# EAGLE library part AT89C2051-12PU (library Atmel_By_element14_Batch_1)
Microcontroller
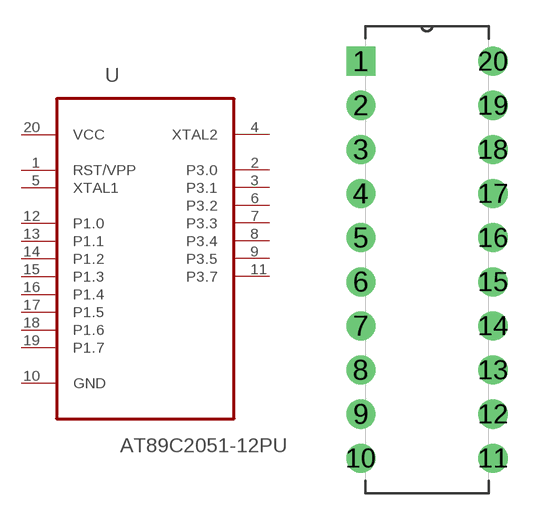
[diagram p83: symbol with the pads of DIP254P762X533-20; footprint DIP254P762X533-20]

Designator prefix U

## AT89C2051-12PU (MPN: AT89C2051-12PU; OC_FARNELL: 1699389; OC_NEWARK: 68T4860; PACKAGE: DIP-20; SUPPLIER: ATMEL)  [DIP254P762X533-20]
1  RST/VPP  in
2  P3.0
3  P3.1
4  XTAL2  out
5  XTAL1  in
6  P3.2
7  P3.3
8  P3.4
9  P3.5
10  GND  pas
11  P3.7
12  P1.0
13  P1.1
14  P1.2
15  P1.3  nc
16  P1.4
17  P1.5
18  P1.6
19  P1.7
20  VCC  pwr

## Footprint DIP254P762X533-20 (pad centres in mm)
drill 1.118 square: 1 -7.62,22.86
drill 1.118: 2 -7.62,20.32; 3 -7.62,17.78; 4 -7.62,15.24; 5 -7.62,12.7; 6 -7.62,10.16; 7 -7.62,7.62; 8 -7.62,5.08; 9 -7.62,2.54; 10 -7.62,0; 11 0,0; 12 0,2.54; 13 0,5.08; 14 0,7.62; 15 0,10.16; 16 0,12.7; 17 0,15.24; 18 0,17.78; 19 0,20.32; 20 0,22.86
